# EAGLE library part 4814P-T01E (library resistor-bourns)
BOURNS RESISTOR NETWORK
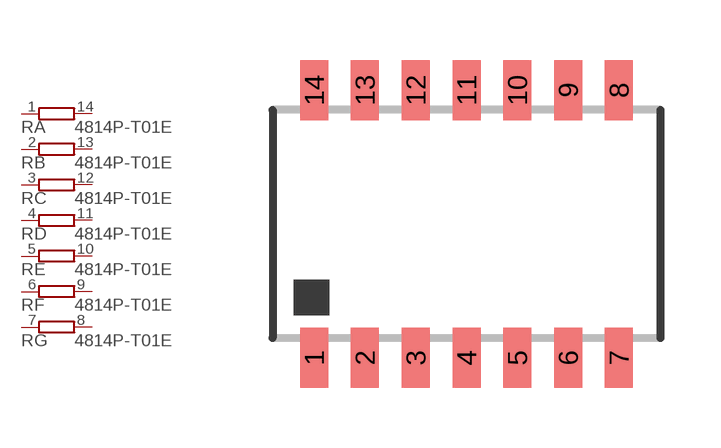
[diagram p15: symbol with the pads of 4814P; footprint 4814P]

Designator prefix R; gates A=R1NV B=R1NV C=R1NV D=R1NV E=R1NV F=R1NV G=R1NV

## 4814P-T01E (OC_FARNELL: unknown; OC_NEWARK: unknown)  [4814P]
1  A:1  pas
2  B:1  pas
3  C:1  pas
4  D:1  pas
5  E:1  pas
6  F:1  pas
7  G:1  pas
8  G:2  pas
9  F:2  pas
10  E:2  pas
11  D:2  pas
12  C:2  pas
13  B:2  pas
14  A:2  pas

## Footprint 4814P (pad centres in mm)
BOURNS RESISTOR NETWORK
smd 0.7 x 1.5: 1 -3.81,-3.346; 2 -2.54,-3.346; 3 -1.27,-3.346; 4 0,-3.346; 5 1.27,-3.346; 6 2.54,-3.346; 7 3.81,-3.346; 8 3.81,3.346; 9 2.54,3.346; 10 1.27,3.346; 11 0,3.346; 12 -1.27,3.346; 13 -2.54,3.346; 14 -3.81,3.346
